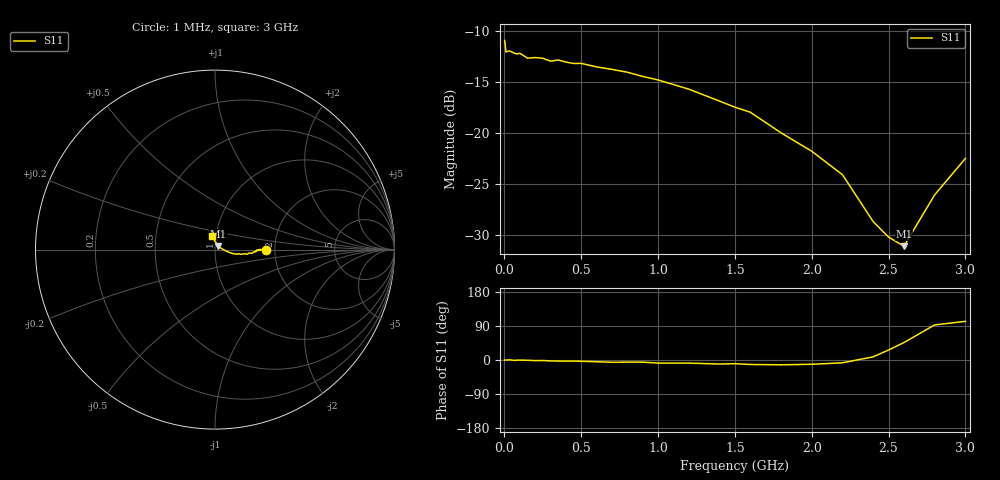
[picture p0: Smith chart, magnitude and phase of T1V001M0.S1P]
! SIEMENS Small Signal Semiconductors
! BAT68-04
! Si Schottky Diode (2 diodes in series, pin 3 open) in SOT23
! IF = 1 mA
! S-Parameters:  August  1994
# GHz  S  MA  R  50
!  f  S11
! GHz  MAG  ANG
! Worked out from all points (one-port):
!   33 points, 1 MHz to 3 GHz, reference 50 ohm
!   lowest |S11| = -31.1 dB at 2.6 GHz (marker M1), VSWR 1.06, Z = 51.9 + j2.09 ohm
!   |S11| at or under -10 dB: start of sweep to end of sweep
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0.001  0.2846 -0.1
0.01  0.2499 -0.2
0.03  0.2529 0.4
0.06  0.2471 -1.2
0.08  0.2444 -0.6
0.1  0.2464 -0.2
0.15  0.233 -0.7
0.25  0.2327 -1.3
0.3  0.2253 -2.5
0.35  0.2284 -2.8
0.4  0.223 -2.9
0.45  0.2195 -2.9
0.5  0.2197 -3.3
0.7  0.2053 -6.0
0.8  0.1988 -5.7
0.9  0.1896 -5.7
1  0.1822 -8.1
1.2  0.1642 -8.2
1.5  0.134 -9.8
1.6  0.1266 -11.8
1.8  0.1003 -12.7
2  0.0815 -11.3
2.2  0.0625 -7.4
2.4  0.0368 8.4
2.5  0.0309 26.3
2.6  0.0279 46.0
2.8  0.0498 92.6
3  0.0751 102.0
